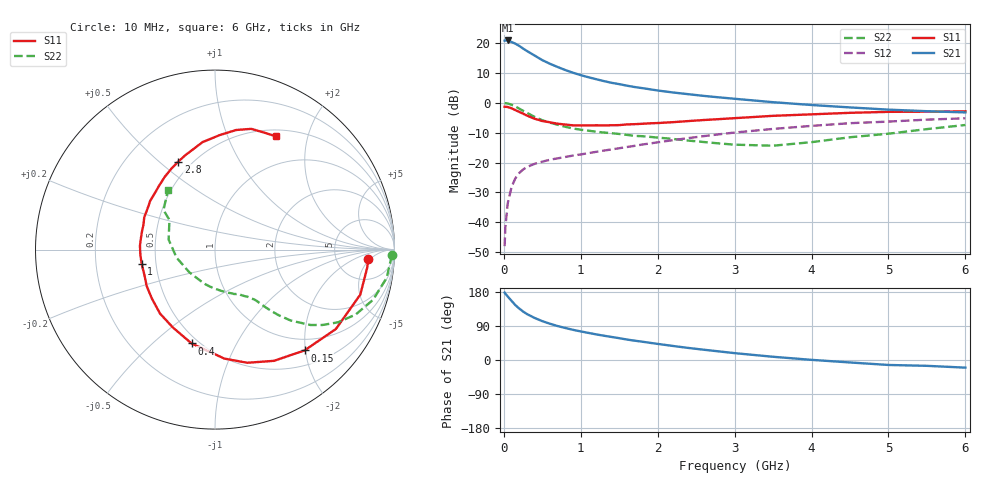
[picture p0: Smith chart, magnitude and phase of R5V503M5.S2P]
! SIEMENS Small Signal Semiconductors
! BFR183
! Si NPN RF Bipolar Junction Transistor in SOT23
! VCE = 0.5 V  IC = 3.5 mA
! Common Emitter S-Parameters:  May  1996
# GHz  S  MA  R  50
!  f  S11  S21  S12  S22
! GHz  MAG  ANG  MAG  ANG  MAG  ANG  MAG  ANG
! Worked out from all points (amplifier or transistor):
!   36 points, 10 MHz to 6 GHz, reference 50 ohm
!   highest |S21| = 20.8 dB at 50 MHz (marker M1)
!   |S21| within 3 dB of that: start of sweep to 268.2 MHz
!   unconditionally stable (mu >= 1): 1.069 GHz to 3.459 GHz
!   at 250 MHz: K = 0.34, MSG = 20.2 dB, |S12| = -22.3 dB
!   at 1.4 GHz: K = 1.10, MAG = 9.2 dB, |S12| = -15.6 dB
!   at 6 GHz: K = 0.98, MSG = 1.0 dB, |S12| = -5.2 dB
!   S11 on the Smith chart (normalised r, x): 10 MHz: 11, -4; 150 MHz: 0.77, -1.98; 400 MHz: 0.46, -0.67; 1 GHz: 0.42, -0.08; 2.8 GHz: 0.42, +0.58; 6 GHz: 0.58, +1.51
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0.01  0.8567 -3.4  10.87 177.9  0.004 87.8  0.9861 -1.8
0.02  0.8537 -6.9  10.95 175.0  0.0084 84.9  0.9802 -3.7
0.05  0.8475 -17.2  10.96 167.6  0.0206 80.5  0.9694 -9.3
0.1  0.8059 -33.3  10.34 156.2  0.0389 72.4  0.9243 -17.6
0.15  0.7513 -48.4  9.676 144.7  0.0546 65.3  0.863 -24.8
0.2  0.7013 -62.1  8.892 135.9  0.0667 59.6  0.7959 -30.6
0.25  0.6556 -74.1  8.025 128.0  0.0764 54.8  0.7321 -35.0
0.3  0.6094 -85.1  7.309 121.3  0.084 51.8  0.6777 -38.3
0.4  0.539 -104.0  6.128 111.0  0.095 47.2  0.5788 -43.1
0.5  0.4935 -118.3  5.139 102.5  0.1032 45.0  0.5086 -45.9
0.6  0.4701 -130.6  4.463 95.7  0.1114 43.7  0.4633 -47.5
0.7  0.4449 -142.3  3.943 89.5  0.1174 43.2  0.427 -48.8
0.8  0.4311 -152.1  3.507 84.4  0.1239 43.4  0.3955 -49.9
1  0.4162 -168.8  2.884 75.4  0.1365 44.2  0.3533 -51.8
1.1  0.4168 -176.1  2.661 71.5  0.1436 44.5  0.3399 -53.3
1.6  0.4332 155.5  1.923 54.0  0.1816 45.8  0.2896 -60.5
2.2  0.4725 131.3  1.48 37.0  0.2367 44.7  0.2477 -74.7
2.8  0.531 112.7  1.226 22.6  0.2963 40.4  0.2084 -97.5
3.5  0.6028 96.6  1.019 8.5  0.3644 32.5  0.1909 -138.5
4.5  0.6765 80.0  0.833 -6.5  0.4542 20.0  0.2643 167.8
5.5  0.7073 67.2  0.72 -15.4  0.5207 8.2  0.3616 142.5
6  0.7162 61.8  0.687 -20.2  0.5485 0.4  0.4238 128.2
